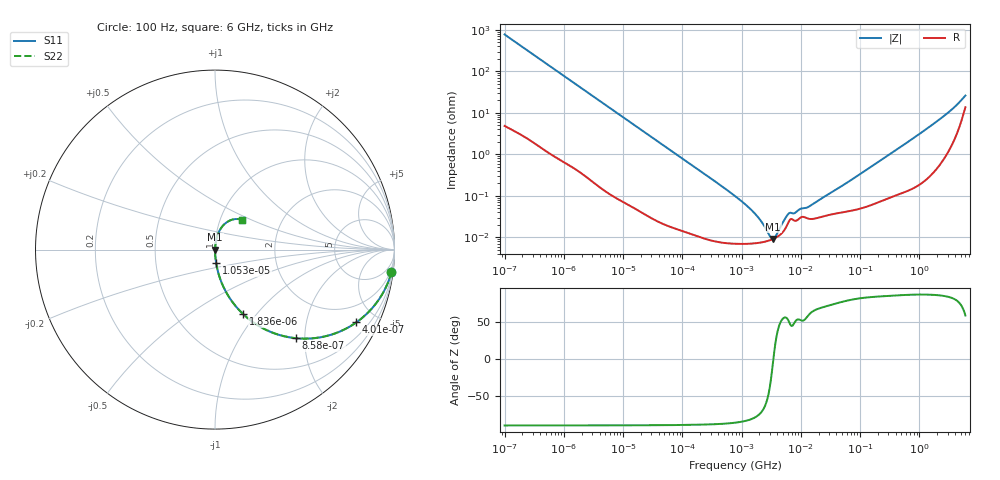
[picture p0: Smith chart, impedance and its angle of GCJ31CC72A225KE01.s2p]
!Murata Part Number: GCJ31CC72A225KE01
!These Parameters are Measured in Series Mode Connection
!Data Generated on Mar 13, 2026
!  o--ll--o
!Port1  Port2
!  o------o
!Operation Temp=25[degC], DC Bias Voltage=0[V]
!Freq. Start=100[Hz] Stop=6[GHz] 401[Steps]
# Hz S RI R 50
!Freq.(Hz) S11(Real) S11(Imag) S21(Real) S21(Imag) S12(Real) S12(Imag) S22(Real) S22(Imag)
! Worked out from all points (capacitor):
!   401 points, 100 Hz to 6 GHz, reference 50 ohm
!   read as one part in series: C = 2.06 uF near 109 Hz
!   lowest |Z| = 9.17 mohm at 3.394 MHz (marker M1)
!   series resonance near 3.447 MHz, so ESL is about 1 nH
!   S11 on the Smith chart (normalised r, x): 100 Hz: 1, -15; 401 Hz: 1.03, -3.88; 858 Hz: 1.01, -1.82; 1.836 kHz: 1.01, -0.85; 10.53 kHz: 1.00, -0.15; 6 GHz: 1.27, +0.44
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100  0.9827 -0.1273  0.0173 0.1273  0.0173 0.1273  0.9827 -0.1273
224  0.9212 -0.2658  0.0788 0.2658  0.0788 0.2658  0.9212 -0.2658
401  0.788 -0.405  0.212 0.405  0.212 0.405  0.788 -0.405
600  0.6265 -0.4799  0.3735 0.4799  0.3735 0.4799  0.6265 -0.4799
858  0.4526 -0.4937  0.5474 0.4937  0.5474 0.4937  0.4526 -0.4937
1836  0.156 -0.3585  0.844 0.3585  0.844 0.3585  0.156 -0.3585
2008  0.1342 -0.3365  0.8658 0.3365  0.8658 0.3365  0.1342 -0.3365
3931  0.0399 -0.1917  0.9601 0.1917  0.9601 0.1917  0.0399 -0.1917
10527  0.00627 -0.0745  0.9937 0.0745  0.9937 0.0745  0.00627 -0.0745
40335  0.000623 -0.0197  0.9994 0.0197  0.9994 0.0197  0.000623 -0.0197
774597  7.14e-05 -0.000992  0.9999 0.000992  0.9999 0.000992  7.14e-05 -0.000992
1658239  7.24e-05 -0.000376  0.9999 0.000376  0.9999 0.000376  7.24e-05 -0.000376
2169299  7.61e-05 -0.000227  0.9999 0.000227  0.9999 0.000227  7.61e-05 -0.000227
2967816  8.5e-05 -7.15e-05  0.9999 7.15e-05  0.9999 7.15e-05  8.5e-05 -7.15e-05
3394479  9.14e-05 -7.3e-06  0.9999 7.3e-06  0.9999 7.3e-06  9.14e-05 -7.3e-06
3882480  0.000101 5.78e-05  0.9999 -5.78e-05  0.9999 -5.78e-05  0.000101 5.78e-05
6075234  0.000219 0.000288  0.9998 -0.000288  0.9998 -0.000288  0.000219 0.000288
1.555665e7  0.000279 0.000556  0.9997 -0.000556  0.9997 -0.000556  0.000279 0.000556
3.124326e8  0.000991 0.00986  0.999 -0.00986  0.999 -0.00986  0.000991 0.00986
3.065283e9  0.0209 0.0974  0.9791 -0.0974  0.9791 -0.0974  0.0209 0.0974
4.385646e9  0.0541 0.1433  0.9459 -0.1433  0.9459 -0.1433  0.0541 0.1433
6e9  0.1523 0.1653  0.8477 -0.1653  0.8477 -0.1653  0.1523 0.1653
